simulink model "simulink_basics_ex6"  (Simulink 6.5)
settings: Solver=ode3  StartTime=0.0  StopTime=Tstop  FixedStep=Tsample  RelTol=1e-3
PreLoadFcn:
  | simulink_basics_ex5_ini
InitFcn:
  | simulink_basics_ex5_ini
StopFcn:
  | simulink_basics_ex5_plot

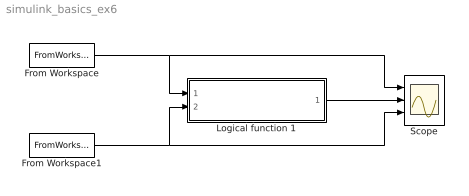
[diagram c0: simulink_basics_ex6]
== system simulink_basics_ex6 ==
  From Workspace : FromWorkspace  VariableName=siminA  SampleTime=0  OutputAfterFinalValue=Holding final value
  From Workspace1 : FromWorkspace  VariableName=siminB  SampleTime=0  OutputAfterFinalValue=Holding final value
  Logical function 1 : Subsystem
  Scope : Scope  NumInputPorts=3
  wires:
  From Workspace/1 -> Logical function 1/1(A), Scope/1
  From Workspace1/1 -> Logical function 1/2(B), Scope/3
  Logical function 1/1(y) -> Scope/2

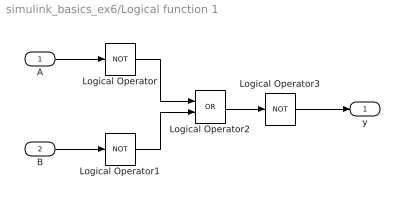
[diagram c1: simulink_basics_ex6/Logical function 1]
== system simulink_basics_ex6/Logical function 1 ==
  A : Inport
  B : Inport  Port=2
  Logical Operator : Logic  Operator=NOT  AllPortsSameDT=off  OutDataTypeMode=Boolean
  Logical Operator1 : Logic  Operator=NOT  AllPortsSameDT=off  OutDataTypeMode=Boolean
  Logical Operator2 : Logic  Operator=OR  AllPortsSameDT=off  OutDataTypeMode=Boolean
  Logical Operator3 : Logic  Operator=NOT  AllPortsSameDT=off  OutDataTypeMode=Boolean
  y : Outport
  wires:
  Logical Operator/1 -> Logical Operator2/1
  Logical Operator1/1 -> Logical Operator2/2
  Logical Operator2/1 -> Logical Operator3/1
  A/1 -> Logical Operator/1
  Logical Operator3/1 -> y/1
  B/1 -> Logical Operator1/1
